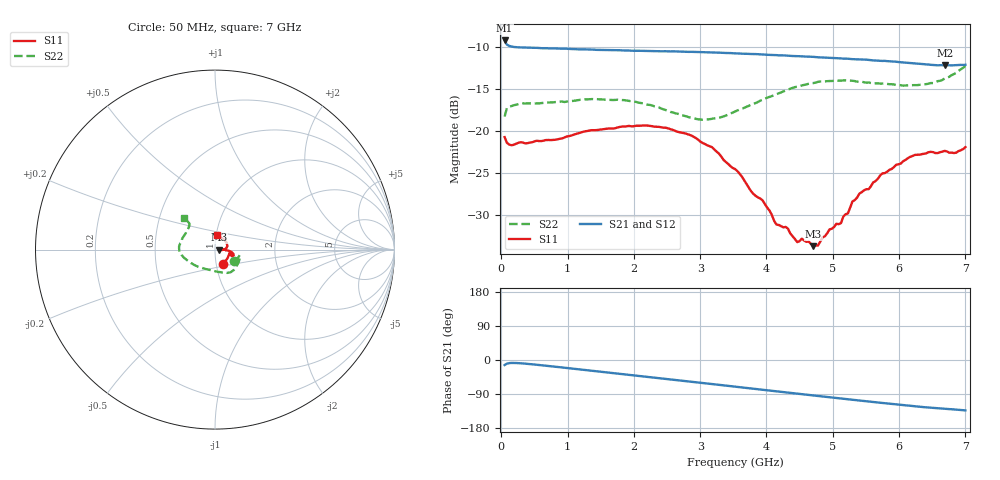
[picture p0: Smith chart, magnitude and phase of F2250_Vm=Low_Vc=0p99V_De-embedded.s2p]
! Integrated Device Technology
! Corporate Headquarters
! 6024 Silver Creek Valley Road
! San Jose, CA 95138  USA
! Phone:  1-408-284-8200
! Toll Free:  1-800-223-1366
! Webpage:  http://www.idt.com/
! Timing and RF Division
! 515 Groton Road, Suite 102
! Westford, MA 01886-6024
! Device:  F2250
! Description: Voltage Variable RF Attenuator
! Frequency:  50.0 -  6000.00 MHz
! Package:  3x3 mm Thin QFN Plastic Package: 16 pin
! Ports:  2 RF, 3 DC
!  Pin  1  = GND
!  Pin  2  = NC
!  Pin  3  = RF1  = Port 1
!  Pin  4  = NC
!  Pin  5  = GND
!  Pin  6  = GND
!  Pin  7  = GND
!  Pin  8  = GND
!  Pin  9  = NC
!  Pin 10  = RF2  = Port 2
!  Pin 11  = NC
!  Pin 12  = GND
!  Pin 13  = GND
!  Pin 14  = VCNTRL
!  Pin 15  = VDD
!  Pin 16  = VMODE
! Vcntrl:  0.990 Volts
! Vmode:  +0.000 Volts
! Vdd:  +3.30  Volts
! Current:  1.185 mA
! Data:  The device was measured on a the F2250 evaluation board which has
!  individual transmission lines to the RF pins.  Data was collected
!  using a calibrated network analyzer.  The evaluation board was
!  de-embedded using a TRL calibration technique.
!  The reference plane is the edge of the package pin.
! Misc:  SN 10
!  Action Tracker AT0258
! Date Measured:  2014-11-26
! Date:  2015-10-15  MJV
! Note:
!  Integrated Device Technology supplies this data as a sample of measured
!  data at the package pin for this product.  Your particular data for this
!  product may vary.
!  Data was taken at 25 degrees C.
!  Integrated Device Technology reserves the right to change this data at anytime.
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# GHz S dB R 50
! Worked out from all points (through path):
!   201 points, 50 MHz to 7 GHz, reference 50 ohm
!   highest |S21| = -9.18 dB at 50 MHz (marker M1); lowest = -12.2 dB at 6.687 GHz (marker M2)
!   group delay of S21, straight-line fit = 52.9 ps
!   lowest |S11| = -33.7 dB at 4.707 GHz (marker M3), VSWR 1.04, Z = 52.1 + j0.0267 ohm
!   |S11| at or under -10 dB: start of sweep to end of sweep
!   |S22| runs from -18.6 to -12.2 dB; largest |S21 - S12| = 0.00082
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0.05  -20.72 -60.3  -9.18 -13.3  -9.18 -13.3  -18.27 -32.4
0.08475  -21.40 -34.7  -9.68 -9.6  -9.68 -9.6  -17.24 -17.8
0.29325  -21.32 -13.5  -10.01 -8.7  -10.02 -8.7  -16.70 -14.6
1.2315  -20.09 -20.2  -10.23 -25.7  -10.23 -25.7  -16.22 -41.6
1.857  -19.46 -18.5  -10.38 -37.6  -10.36 -37.6  -16.30 -55.6
2.37825  -19.49 -14.1  -10.46 -47.6  -10.46 -47.6  -17.18 -69.0
3.0385  -21.42 -7.0  -10.57 -60.6  -10.58 -60.6  -18.64 -101.0
3.525  -24.52 -2.8  -10.72 -70.3  -10.71 -70.3  -17.65 -131.1
3.803  -27.49 -0.6  -10.80 -75.8  -10.78 -75.9  -16.74 -144.7
3.942  -28.27 0.8  -10.86 -78.6  -10.85 -78.6  -16.25 -151.2
4.1505  -31.15 2.1  -10.93 -82.7  -10.92 -82.7  -15.59 -159.2
4.32425  -31.65 3.0  -11.01 -86.0  -11.00 -86.1  -15.03 -164.5
4.46325  -33.25 1.8  -11.05 -88.8  -11.06 -88.8  -14.71 -168.3
4.53275  -32.84 0.9  -11.07 -90.2  -11.06 -90.3  -14.54 -170.4
4.7065  -33.73 0.7  -11.13 -93.6  -11.14 -93.6  -14.26 -174.1
5.1235  -30.98 -4.9  -11.32 -101.7  -11.32 -101.7  -13.98 176.6
5.4015  -27.46 -2.2  -11.44 -106.9  -11.44 -106.9  -14.10 170.1
5.85325  -24.62 4.5  -11.66 -115.3  -11.66 -115.4  -14.40 158.6
6.2355  -22.85 17.7  -11.91 -122.1  -11.91 -122.1  -14.52 146.0
6.68725  -22.36 46.0  -12.16 -128.6  -12.16 -128.6  -13.72 134.4
6.861  -22.57 61.7  -12.13 -130.9  -12.13 -130.9  -13.05 134.2
7  -21.91 80.1  -12.08 -133.0  -12.06 -133.1  -12.22 134.3
